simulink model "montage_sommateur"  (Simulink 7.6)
settings: Solver=ode15s  StartTime=0.0  StopTime=1  MaxStep=0.00002  RelTol=1e-3
StopFcn:
  | load signaux.mat
  | subplot 211
  | plot(x(1,:),x(3,:),x(1,:),x(4,:))
  | axis([0 1 -1.5 2.5])
  | title('montage sommateur')
  | grid
  | 
  | subplot 212
  | plot(x(1,:),x(2,:))
  | grid
  | axis([0 1 -0.2 1.2])
undefined symbols (not defined in the file or in its folder): sigbuilder_block
libraries: fl_lib x14, nesl_utility x4, elec_lib x2

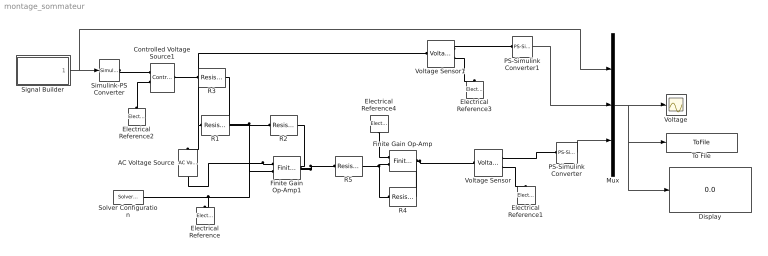
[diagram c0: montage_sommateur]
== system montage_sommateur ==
  AC Voltage Source : fl_lib/Electrical/Electrical Sources/AC Voltage Source  DialogController=NetworkEngine.DynNeDlgSource  SystemSampleTime=-1  amp=1 V  shift=0 rad  omega=1 Hz  i_Log=off  v_Log=off  LocalVarNames=|current|voltage|power  LocalVarDescs=|Current (A)|Voltage (V)|Power (W)  LocalVarLogging=[0 0 0]
  Controlled Voltage Source1 : fl_lib/Electrical/Electrical Sources/Controlled Voltage Source  DialogController=NetworkEngine.DynNeDlgSource  SystemSampleTime=-1  i_Log=off  v_Log=off  LocalVarNames=|current|voltage|power  LocalVarDescs=|Current (A)|Voltage (V)|Power (W)  LocalVarLogging=[0 0 0]
  Display : Display
  Electrical Reference{,1..4} (5 alike) : fl_lib/Electrical/Electrical Elements/Electrical Reference  DialogController=NetworkEngine.DynNeDlgSource  SystemSampleTime=-1  i_Log=off  LocalVarNames=|i  LocalVarDescs=|i  LocalVarLogging=[]
  Finite Gain Op-Amp : elec_lib/Integrated Circuits/Finite Gain Op-Amp  DialogController=NetworkEngine.DynNeDlgSource  SystemSampleTime=-1  A=1000  Rin=1e+06 Ohm  Rout=100 Ohm  Vmin=-15 V  Vmax=15 V  LocalVarNames=|power  LocalVarDescs=|Dissipated power (W)  LocalVarLogging=0
  Finite Gain Op-Amp1 : elec_lib/Integrated Circuits/Finite Gain Op-Amp  DialogController=NetworkEngine.DynNeDlgSource  SystemSampleTime=-1  A=1000  Rin=1e+06 Ohm  Rout=100 Ohm  Vmin=-15 V  Vmax=15 V  LocalVarNames=|power  LocalVarDescs=|Dissipated power (W)  LocalVarLogging=0
  Mux : Mux  Inputs=3
  PS-Simulink Converter : nesl_utility/PS-Simulink Converter  DialogController=NetworkEngine.DynNeUtilDlgSource  SystemSampleTime=-1  PhysicalDomain=network_engine_domain  LeftPortType=input  RightPortType=output  SubClassName=ps_output  Unit=V  AffineConversion=off
  PS-Simulink Converter1 : nesl_utility/PS-Simulink Converter  DialogController=NetworkEngine.DynNeUtilDlgSource  SystemSampleTime=-1  PhysicalDomain=network_engine_domain  LeftPortType=input  RightPortType=output  SubClassName=ps_output  Unit=V  AffineConversion=off
  R{1..5} (5 alike) : fl_lib/Electrical/Electrical Elements/Resistor  DialogController=NetworkEngine.DynNeDlgSource  SystemSampleTime=-1  R=10e3 Ohm  i_Log=off  v_Log=off  LocalVarNames=|current|voltage|power  LocalVarDescs=|Resistor current (A)|Voltage across resistor (V)|Power (W)  LocalVarLogging=[0 0 0]
  Signal Builder : Subsystem  Tag=STV Subsys  LoadFcn=sigbuilder_block('load');  StartFcn=sigbuilder_block('start');  StopFcn=sigbuilder_block('stop');  ClipboardFcn=sigbuilder_block('clipboard');
  Simulink-PS Converter : nesl_utility/Simulink-PS Converter  DialogController=NetworkEngine.DynNeUtilDlgSource  SystemSampleTime=-1  PhysicalDomain=network_engine_domain  LeftPortType=input  RightPortType=output  SubClassName=ps_input  Unit=1  AffineConversion=off  InputFilterTimeConstant=.001  UdotUserProvided=0
  Solver Configuration : nesl_utility/Solver Configuration  DialogController=NetworkEngine.DynNeUtilDlgSource  SystemSampleTime=-1  PhysicalDomain=network_engine_domain  LeftPortType=input  RightPortType=generic  SubClassName=solver  Accelerate=off  Profile=off  ResidualTolerance=1e-9  MaxNonlinIter=12  MaxModeIter=2  DoFixedCost=off  UseLocalSampling=off  DoDC=off  LinearAlgebra=Sparse  LocalSolverSampleTime=.001  LocalSolverChoice=NE_BACKWARD_EULER_ADVANCER  UseLocalSolver=off
  To File : ToFile  Filename=signaux  MatrixName=x
  Voltage : Scope
  Voltage Sensor : fl_lib/Electrical/Electrical Sensors/Voltage Sensor  DialogController=NetworkEngine.DynNeDlgSource  SystemSampleTime=-1  i1_Log=off  v1_Log=off  LocalVarNames=|i1|v1  LocalVarDescs=|i1|v1  LocalVarLogging=[]
  Voltage Sensor1 : fl_lib/Electrical/Electrical Sensors/Voltage Sensor  DialogController=NetworkEngine.DynNeDlgSource  SystemSampleTime=-1  i1_Log=off  v1_Log=off  LocalVarNames=|i1|v1  LocalVarDescs=|i1|v1  LocalVarLogging=[]
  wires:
  Mux/1 -> Voltage/1, To File/1, Display/1
  Signal Builder/1(Signal 2) -> Simulink-PS Converter/1, Mux/1
  PS-Simulink Converter/1 -> Mux/3
  PS-Simulink Converter1/1 -> Mux/2
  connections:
  Finite Gain Op-Amp1/LConn1 -- Electrical Reference/LConn1 -- Solver Configuration/RConn1 -- AC Voltage Source/RConn1
  Finite Gain Op-Amp1/LConn2 -- R3/RConn1 -- R1/RConn1 -- R2/LConn1
  Finite Gain Op-Amp1/RConn1 -- R2/RConn1 -- R5/LConn1
  Voltage Sensor/RConn2 -- Electrical Reference1/LConn1
  Voltage Sensor/RConn1 -- PS-Simulink Converter/LConn1
  Voltage Sensor1/RConn1 -- PS-Simulink Converter1/LConn1
  Simulink-PS Converter/RConn1 -- Controlled Voltage Source1/RConn1
  Controlled Voltage Source1/LConn1 -- R3/LConn1
  Electrical Reference2/LConn1 -- Controlled Voltage Source1/RConn2
  Electrical Reference4/LConn1 -- Finite Gain Op-Amp/LConn1
  Finite Gain Op-Amp/RConn1 -- Voltage Sensor/LConn1 -- R4/RConn1
  Finite Gain Op-Amp/LConn2 -- R5/RConn1 -- R4/LConn1
  Voltage Sensor1/RConn2 -- Electrical Reference3/LConn1
  R1/LConn1 -- AC Voltage Source/LConn1 -- Voltage Sensor1/LConn1

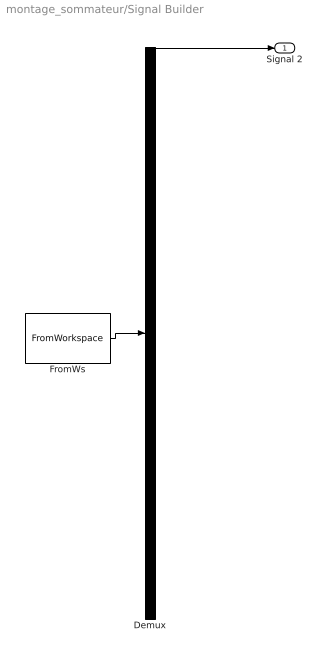
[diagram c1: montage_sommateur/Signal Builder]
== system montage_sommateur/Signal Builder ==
  Demux : Demux  Tag=STV Demux  Outputs=1
  FromWs : FromWorkspace  Tag=STV FromWs  VariableName=tuvar  SampleTime=0  SigBuilderData=DataTag0  VnvData=DataTag1
  Signal 2 : Outport  Tag=STV Outport
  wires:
  FromWs/1 -> Demux/1
  Demux/1 -> Signal 2/1
